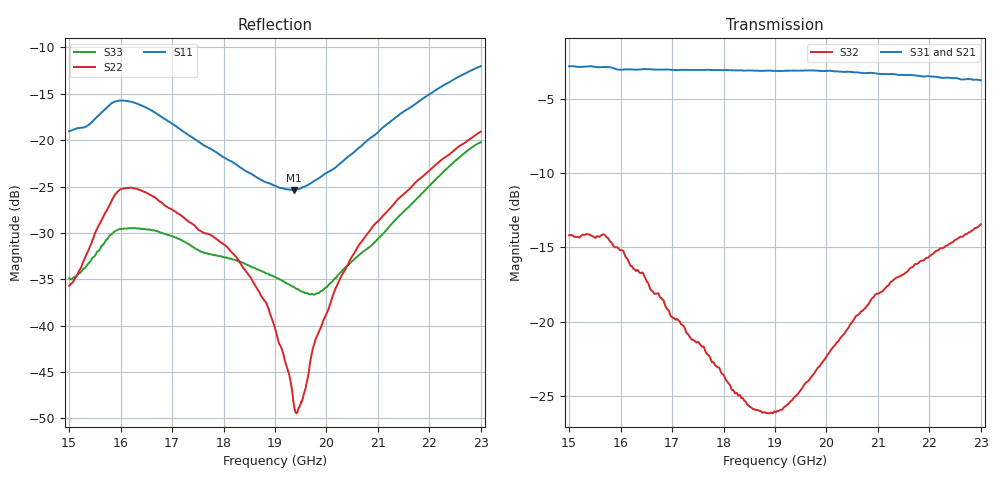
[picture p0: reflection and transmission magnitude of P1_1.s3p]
!The following data was pulled from an Agilent PNA
!This sNp file was generated from the data in the RF Test software
!NOTE:  Smoothing/Math/Corrections applied on any given trace ARE included in the data saved here
# MHz S dB R 50
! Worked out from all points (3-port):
!   1601 points, 15 GHz to 23 GHz, reference 50 ohm
!   strongest paths, dB at 15 GHz, 17 GHz, 19 GHz, 21 GHz, 23 GHz:
!     S31: -2.8, -3.0, -3.1, -3.3, -3.7
!     S21: -3.1, -2.9, -3.1, -3.3, -3.8
!     S32: -14.2, -19.7, -26.1, -18.1, -13.4
!   lowest |S11| = -25.4 dB at 19.37 GHz (marker M1), VSWR 1.11, Z = 49.5 - j5.36 ohm
!   |S11| at or under -10 dB: start of sweep to end of sweep
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15000  -19.04 46.9  -3.08 -168.3  -2.88 -169.3
       -3.05 -168.1  -35.70 123.9  -14.23 150.5
       -2.80 -169.0  -14.18 150.5  -34.91 -160.5
15615  -17.10 50.6  -2.82 -175.9  -2.94 -178.9
       -2.79 -176.1  -28.77 104.9  -14.26 136.3
       -2.85 -178.8  -14.20 136.6  -31.55 125.2
15690  -16.71 49.2  -2.76 -177.2  -2.95 10.5
       -2.77 -177.0  -27.96 101.4  -14.27 133.0
       -2.84 -10.5  -14.15 133.0  -31.02 114.3
15785  -16.20 46.1  -2.75 -179.0  -3.00 178.2
       -2.70 -178.4  -27.01 95.6  -14.64 129.1
       -2.85 178.4  -14.54 128.7  -30.31 100.3
15855  -15.92 42.8  -2.76 -10.8  -3.08 177.3
       -2.64 -10.3  -26.23 90.1  -14.90 126.9
       -2.92 177.1  -14.87 126.3  -29.96 90.6
15940  -15.76 38.8  -2.75 178.5  -3.12 176.3
       -2.66 178.6  -25.56 81.9  -15.01 123.7
       -3.01 176.3  -15.00 123.6  -29.68 79.1
19000  -24.91 -67.8  -3.18 136.7  -3.12 136.6
       -3.14 136.1  -40.28 12.1  -26.03 11.3
       -3.10 135.5  -26.06 10.7  -34.76 -55.7
19370  -25.36 -91.8  -3.14 131.3  -3.08 131.0
       -3.13 131.0  -48.73 55.0  -25.08 -13.8
       -3.09 130.5  -25.11 -14.0  -35.83 -81.4
20630  -20.82 -156.1  -3.26 112.1  -3.24 111.5
       -3.23 112.3  -31.28 146.7  -19.49 -75.9
       -3.22 111.7  -19.50 -76.0  -32.40 -166.9
23000  -12.02 152.6  -3.80 77.5  -3.73 77.1
       -3.76 77.6  -19.08 127.7  -13.37 -131.1
       -3.74 77.0  -13.44 -131.4  -20.21 144.2
